(* Logix 5000 Rung export; software revision 16.03 *)

MODULES
   MNETC : vendor None type None code None
   Local : vendor None type None code None
END_MODULES

TYPE MNetCConnectionInput :
STRUCT
   Data : INT[62];   // Block Transfer Array Size [62] or [122] or [242]
END_STRUCT
END_TYPE

TYPE MNetCInitOutData :   // Used to bring the Module into a known state after a restart operation.
STRUCT
   InitOutBlkIDLim : INT;   // Block Index Limit for ReadData size of the array
END_STRUCT
END_TYPE

TYPE MnetCCmdControl :
STRUCT
   CmdCntReqClientID : INT;   // Block5000 Client IDentification by Index number 0 to 29
   CmdCntReqCMDqty : INT;   // Block5000 command quantity
   CmdCntReqCMDindex : INT[16];   // Contains index in the command list for the 1st command to be entered into Command queue
   WriteCmdBits : INT[30];   // This is for 30 Clients with 16 commands each.
   CmdBitsTrigger : BOOL;   // Activates the Selected Write Command Bits
END_STRUCT
END_TYPE

TYPE MNetCDATA :
STRUCT
   ReadData : INT[480];
   WriteData : INT[480];
END_STRUCT
END_TYPE

TYPE MNetCCONTROL :
STRUCT
   BootTimer : TIMER;
   ColdBoot : BOOL;   // Hardware reset of the Module
   WarmBoot : BOOL;   // Configuration data reset in the Module.
   EventCmd : MNetCEventCmd[1];
   EventCmdTrigger : BOOL;
   EventCmdPending : BOOL;   // Halts rung until Module is ready.
   CmdControl : MnetCCmdControl;
   CmdControlPending : BOOL;   // Halts rung until Module is ready.
   CmdControlTrigger : BOOL;
   IPAdressControl : MNetCIPAddress;
   CmdBitPending : BOOL;   // Halts rung until Module is ready.
   CmdBitTrigger : BOOL;
END_STRUCT
END_TYPE

TYPE MNetCCONFIG :
STRUCT
   BlockTransferSize : INT;   // Determines Register quantity to move across the Backplane
END_STRUCT
END_TYPE

TYPE MNetCIPAddress :   // Dynamicaly Alterable TCP/IP address for MNETC module. Block 9990 and 9991
STRUCT
   GetIPAddress : BOOL;   // Gets IP address
   GetIP : INT[4];   // Get IP
   GetIPAddressPending : BOOL;   // Halts rung until Module is ready.
   SetIPAddress : BOOL;   // Sets IP address
   SetIP : INT[4];   // Set IP
   SetIPAddrPending : BOOL;   // Halts rung until Module is ready.
   WriteIPAddressAck : INT[4];   // Module's response to Setting IP Address
END_STRUCT
END_TYPE

TYPE MNetCConnectionOutput :
STRUCT
   Data : INT[61];   // Block Transfer Array Size [61] or [121] or [241]
END_STRUCT
END_TYPE

TYPE MNetCSTATUS :   // This status data is returned on each read block and can be used to detect proper module operation.
STRUCT
   PassCnt : INT;   // Program cycle counter
   Block : MNetCBlockStats;   // Block transfer statistics
   MnetServer : MNetCPortStats;   // MNet server status data
   MBAPServer : MNetCPortStats;   // MBAP server status data
   StatReqClientID : INT;   // Block3000 Client IDentification by Index number 0 to 29
   CmdBits : INT[30];
   ClientStats : MNetCPortStats[30];   // Client status data
   ClientStatsPending : BOOL;   // Halts rung until Module is ready.
   ClientStatsTrigger : BOOL;   // Get Client Status
   CmdErrorList : INT[16];   // Cmd Error List
END_STRUCT
END_TYPE

TYPE MNetCModuleDef :
STRUCT
   CONFIG : MNetCCONFIG;
   DATA : MNetCDATA;
   CONTROL : MNetCCONTROL;
   STATUS : MNetCSTATUS;
   UTIL : MNetCUTIL;
END_STRUCT
END_TYPE

TYPE MNetCUTIL :
STRUCT
   ReadDataSizeGet : INT;   // Gets ReadData Array Length.
   WriteDataSizeGet : INT;   // Gets WriteData Array Length.
   ReadDataBlkCount : INT;   // holds the value of the Block Counts of the Read Data Array.
   WriteDataBlkCount : INT;   // holds the value of the Block Counts of the Write Data Array.
   RBTSremainder : INT;   // The remainder of the 60, 120 or 240 block to transfer.
   WBTSremainder : INT;   // The remainder of the 60, 120 or 240 block to transfer.
   LastRead : INT;   // Index of last read block
   LastWrite : INT;   // Index of last write block
   BlockIndex : INT;   // Computed block offset for data table
   StatusIndex : INT;   // Computed block offset for status data
   InitOutputData : MNetCInitOutData;
END_STRUCT
END_TYPE

TYPE MNetCPortStats :   // This object is used to store the port statistics for an MVI69-MNet port.
STRUCT
   CmdReq : INT;   // Total number of command list requests sent
   CmdResp : INT;   // Total number of command list responses received
   CmdErr : INT;   // Total number of command list errors
   Requests : INT;   // Total number of requests for port
   Responses : INT;   // Total number of responses for port
   ErrSent : INT;   // Total number of errors sent
   ErrRec : INT;   // Total number of errors received
   CfgErrWord : INT;   // Configuration Error Word
   CurErr : INT;   // Current Error code
   LastErr : INT;   // Last recorded error code
END_STRUCT
END_TYPE

TYPE MNetCBlockStats :   // This object is used to store the block transfer statistics for the MVI69-MNet module.
STRUCT
   Read : INT;   // Total number of read block transfers
   Write : INT;   // Total number of write block transfers
   Parse : INT;   // Total number of blocks parsed
   Event : INT;   // Total number of event blocks received
   Cmd : INT;   // Total number of command blocks received
   Err : INT;   // Total number of block transfer errors
END_STRUCT
END_TYPE

TYPE MNetCEventCmd :   // Data structure to use for Event message generation.
STRUCT
   IP0 : INT;   // TCP/IP-0 address for MNETC module
   IP1 : INT;   // TCP/IP-1 address for MNETC module
   IP2 : INT;   // TCP/IP-2 address for MNETC module
   IP3 : INT;   // TCP/IP-3 address for MNETC module
   ServPort : INT;   // TCP Service Port number (0-65535), 502 for MBAP, 2000 for MNET
   Node : INT;   // Modbus slave node address (0 to 247)
   DBAddress : INT;   // Module internal database to use with message
   Count : INT;   // Register or data point count
   Swap : INT;   // Swap code to use with functions 3 and 4
   Function : INT;   // Modbus function code for message
   Address : INT;   // Address to interface with in device
   EvntCmdClientID : INT;   // Block2000 Client IDentification by Index number 0 to 29
END_STRUCT
END_TYPE

ADD_ON_INSTRUCTION AOI69MNETC   (* revision 1.3, vendor ProSoft Technology Inc. *)
// Add On instruction interface between the CompactLogix backplane and the MVI69-MNETC module.
// Revision note:
// v1.3 - Initialize output data block now supports flexible read and write data array sizing.
VAR_IN_OUT
   Connection_Input : MNetCConnectionInput; {required}
   Connection_Output : MNetCConnectionOutput; {required}
   MNETC : MNetCModuleDef; {required}
END_VAR

ROUTINE Logic   (* ladder *)
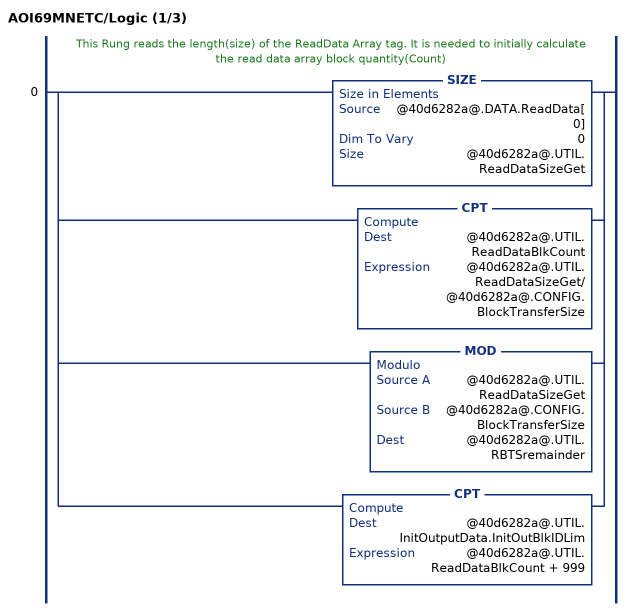
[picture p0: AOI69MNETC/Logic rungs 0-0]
   // This Rung reads the length(size) of the ReadData Array tag. It is needed to initially calculate the read data array block quantity(Count)
   0: [SIZE(@40d6282a@.DATA.ReadData[0],0,@40d6282a@.UTIL.ReadDataSizeGet) ,CPT(@40d6282a@.UTIL.ReadDataBlkCount,@40d6282a@.UTIL.ReadDataSizeGet/@40d6282a@.CONFIG.BlockTransferSize) ,MOD(@40d6282a@.UTIL.ReadDataSizeGet,@40d6282a@.CONFIG.BlockTransferSize,@40d6282a@.UTIL.RBTSremainder) ,CPT(@40d6282a@.UTIL.InitOutputData.InitOutBlkIDLim,@40d6282a@.UTIL.ReadDataBlkCount + 999) ];
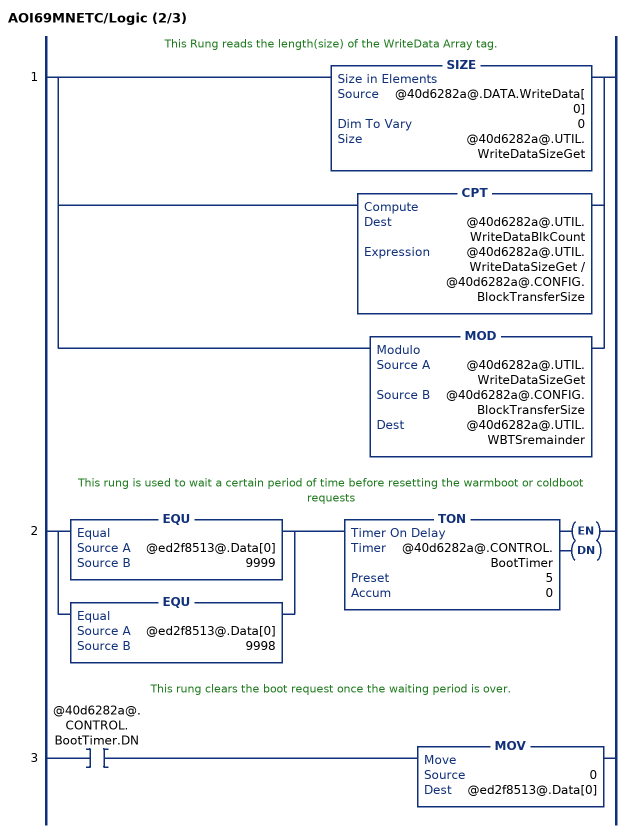
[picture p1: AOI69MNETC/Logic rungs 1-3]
   // This Rung reads the length(size) of the WriteData Array tag.
   1: [SIZE(@40d6282a@.DATA.WriteData[0],0,@40d6282a@.UTIL.WriteDataSizeGet) ,CPT(@40d6282a@.UTIL.WriteDataBlkCount,@40d6282a@.UTIL.WriteDataSizeGet / @40d6282a@.CONFIG.BlockTransferSize) ,MOD(@40d6282a@.UTIL.WriteDataSizeGet,@40d6282a@.CONFIG.BlockTransferSize,@40d6282a@.UTIL.WBTSremainder) ];
   // This rung is used to wait a certain period of time before resetting the warmboot or coldboot requests
   2: [EQU(@ed2f8513@.Data[0],9999) ,EQU(@ed2f8513@.Data[0],9998) ]TON(@40d6282a@.CONTROL.BootTimer,5,0);
   // This rung clears the boot request once the waiting period is over.
   3: XIC(@40d6282a@.CONTROL.BootTimer.DN)MOV(0,@ed2f8513@.Data[0]);
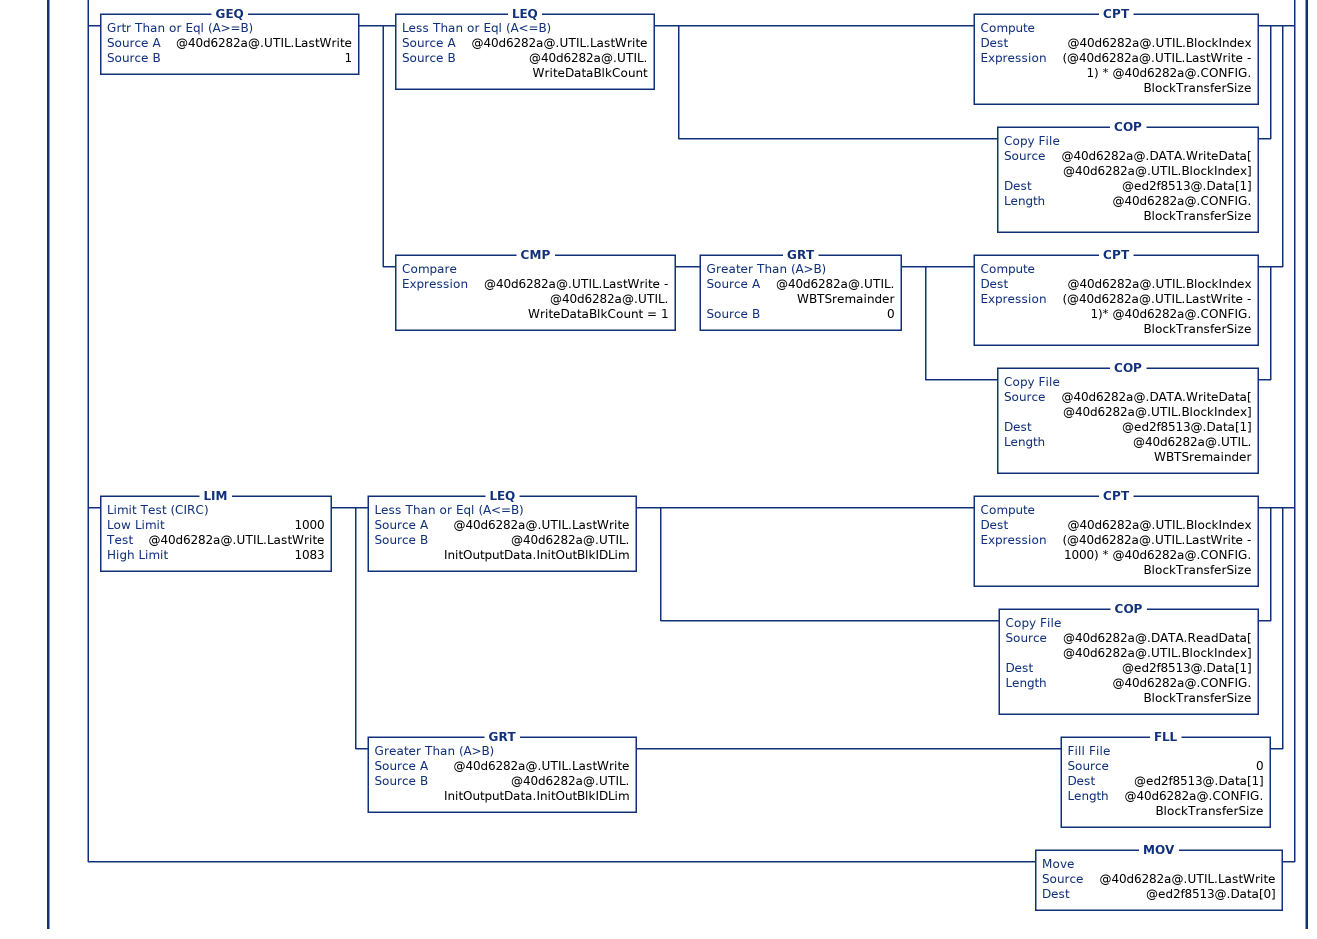
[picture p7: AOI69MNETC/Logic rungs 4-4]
   // This rung is used to check for a new read block from the MVI56-MNETC module in slot 1.  If new data is available, the LastRead and word[0] will not be equal.  This will force the program to call the ReadData subroutine to process the new data received.  After the new data is placed in the Modbus Data Table, the program will send new data to the module using the WriteData subroutine.
   4: NEQ(@f68caed0@.Data[0],@40d6282a@.UTIL.LastRead)[MOV(@f68caed0@.Data[0],@40d6282a@.UTIL.LastRead) ,GEQ(@40d6282a@.UTIL.LastRead,1) [LEQ(@40d6282a@.UTIL.LastRead,@40d6282a@.UTIL.ReadDataBlkCount) [CPT(@40d6282a@.UTIL.BlockIndex,(@40d6282a@.UTIL.LastRead-1)*@40d6282a@.CONFIG.BlockTransferSize) ,COP(@f68caed0@.Data[2],@40d6282a@.DATA.ReadData[@40d6282a@.UTIL.BlockIndex],@40d6282a@.CONFIG.BlockTransferSize) ] ,CMP(@40d6282a@.UTIL.LastRead - @40d6282a@.UTIL.ReadDataBlkCount = 1) GRT(@40d6282a@.UTIL.RBTSremainder,0) [CPT(@40d6282a@.UTIL.BlockIndex,(@40d6282a@.UTIL.LastRead - 1) * @40d6282a@.CONFIG.BlockTransferSize) ,COP(@f68caed0@.Data[2],@40d6282a@.DATA.ReadData[@40d6282a@.UTIL.BlockIndex],@40d6282a@.UTIL.RBTSremainder) ] ] ,[EQU(-1,@40d6282a@.UTIL.LastRead) ,EQU(0,@40d6282a@.UTIL.LastRead) ] [COP(@f68caed0@.Data[2],@40d6282a@.STATUS.PassCnt,1) ,COP(@f68caed0@.Data[3],@40d6282a@.STATUS.Block.Read,6) ,COP(@f68caed0@.Data[9],@40d6282a@.STATUS.CmdBits[0],30) ] ,LIM(2000,@40d6282a@.UTIL.LastRead,2029) EQU(@f68caed0@.Data[2],1) OTU(@40d6282a@.CONTROL.EventCmdPending) ,LIM(3000,@40d6282a@.UTIL.LastRead,3029) [COP(@f68caed0@.Data[2],@40d6282a@.STATUS.ClientStats[@40d6282a@.STATUS.StatReqClientID].CmdReq,10) ,COP(@f68caed0@.Data[12],@40d6282a@.STATUS.CmdErrorList[0],16) ,OTU(@40d6282a@.STATUS.ClientStatsPending) ] ,LIM(5000,@40d6282a@.UTIL.LastRead,5016) LIM(1,@f68caed0@.Data[2],16) OTU(@40d6282a@.CONTROL.CmdControlPending) ,EQU(@40d6282a@.UTIL.LastRead,9990) [COP(@f68caed0@.Data[2],@40d6282a@.CONTROL.IPAdressControl.WriteIPAddressAck[0],4) ,OTU(@40d6282a@.CONTROL.IPAdressControl.SetIPAddrPending) ] ,EQU(@40d6282a@.UTIL.LastRead,9991) [COP(@f68caed0@.Data[2],@40d6282a@.CONTROL.IPAdressControl.GetIP[0],4) ,OTU(@40d6282a@.CONTROL.IPAdressControl.GetIPAddressPending) ] ,MOV(@f68caed0@.Data[1],@40d6282a@.UTIL.LastWrite) ,LIM(1000,@40d6282a@.UTIL.LastWrite,1008) [CPT(@40d6282a@.UTIL.BlockIndex,(@40d6282a@.UTIL.LastWrite - 1000) * @40d6282a@.CONFIG.BlockTransferSize) ,COP(@40d6282a@.DATA.ReadData[@40d6282a@.UTIL.BlockIndex],@ed2f8513@.Data[1],@40d6282a@.CONFIG.BlockTransferSize) ] ,XIC(@40d6282a@.CONTROL.WarmBoot) [MOV(9998,@40d6282a@.UTIL.LastWrite) ,OTU(@40d6282a@.CONTROL.WarmBoot) ] ,XIC(@40d6282a@.CONTROL.ColdBoot) [MOV(9999,@40d6282a@.UTIL.LastWrite) ,OTU(@40d6282a@.CONTROL.ColdBoot) ] ,XIC(@40d6282a@.CONTROL.EventCmdTrigger) XIO(@40d6282a@.CONTROL.EventCmdPending) [COP(@40d6282a@.CONTROL.EventCmd[0].IP0,@ed2f8513@.Data[1],11) ,LIM(0,@40d6282a@.CONTROL.EventCmd[0].EvntCmdClientID,29) ADD(2000,@40d6282a@.CONTROL.EventCmd[0].EvntCmdClientID,@40d6282a@.UTIL.LastWrite) ,OTU(@40d6282a@.CONTROL.EventCmdTrigger) ,OTL(@40d6282a@.CONTROL.EventCmdPending) ] ,XIC(@40d6282a@.STATUS.ClientStatsTrigger) XIO(@40d6282a@.STATUS.ClientStatsPending) [LIM(0,@40d6282a@.STATUS.StatReqClientID,29) ADD(3000,@40d6282a@.STATUS.StatReqClientID,@40d6282a@.UTIL.LastWrite) ,OTL(@40d6282a@.STATUS.ClientStatsPending) ,OTU(@40d6282a@.STATUS.ClientStatsTrigger) ] ,XIC(@40d6282a@.CONTROL.CmdControlTrigger) XIO(@40d6282a@.CONTROL.CmdControlPending) [LIM(0,@40d6282a@.CONTROL.CmdControl.CmdCntReqClientID,29) MOV(@40d6282a@.CONTROL.CmdControl.CmdCntReqClientID,@ed2f8513@.Data[1]) ,COP(@40d6282a@.CONTROL.CmdControl.CmdCntReqCMDindex[0],@ed2f8513@.Data[2],16) ,LIM(1,@40d6282a@.CONTROL.CmdControl.CmdCntReqCMDqty,16) ADD(5000,@40d6282a@.CONTROL.CmdControl.CmdCntReqCMDqty,@40d6282a@.UTIL.LastWrite) ,OTL(@40d6282a@.CONTROL.CmdControlPending) ,OTU(@40d6282a@.CONTROL.CmdControlTrigger) ] ,[EQU(@40d6282a@.UTIL.LastWrite,0) ,EQU(@40d6282a@.UTIL.LastWrite,-1) ,XIC(@40d6282a@.CONTROL.CmdControl.CmdBitsTrigger) MOV(0,@40d6282a@.UTIL.LastWrite) ] [COP(@40d6282a@.CONTROL.CmdControl.WriteCmdBits[0],@ed2f8513@.Data[1],30) ,OTU(@40d6282a@.CONTROL.CmdControl.CmdBitsTrigger) ] ,XIC(@40d6282a@.CONTROL.IPAdressControl.SetIPAddress) XIO(@40d6282a@.CONTROL.IPAdressControl.SetIPAddrPending) [MOV(9990,@40d6282a@.UTIL.LastWrite) ,COP(@40d6282a@.CONTROL.IPAdressControl.SetIP[0],@ed2f8513@.Data[1],4) ,OTL(@40d6282a@.CONTROL.IPAdressControl.SetIPAddrPending) ,OTU(@40d6282a@.CONTROL.IPAdressControl.SetIPAddress) ] ,XIC(@40d6282a@.CONTROL.IPAdressControl.GetIPAddress) XIO(@40d6282a@.CONTROL.IPAdressControl.GetIPAddressPending) [MOV(9991,@40d6282a@.UTIL.LastWrite) ,OTL(@40d6282a@.CONTROL.IPAdressControl.GetIPAddressPending) ,OTU(@40d6282a@.CONTROL.IPAdressControl.GetIPAddress) ] ,GEQ(@40d6282a@.UTIL.LastWrite,1) [LEQ(@40d6282a@.UTIL.LastWrite,@40d6282a@.UTIL.WriteDataBlkCount) [CPT(@40d6282a@.UTIL.BlockIndex,(@40d6282a@.UTIL.LastWrite - 1) * @40d6282a@.CONFIG.BlockTransferSize) ,COP(@40d6282a@.DATA.WriteData[@40d6282a@.UTIL.BlockIndex],@ed2f8513@.Data[1],@40d6282a@.CONFIG.BlockTransferSize) ] ,CMP(@40d6282a@.UTIL.LastWrite - @40d6282a@.UTIL.WriteDataBlkCount = 1) GRT(@40d6282a@.UTIL.WBTSremainder,0) [CPT(@40d6282a@.UTIL.BlockIndex,(@40d6282a@.UTIL.LastWrite - 1)* @40d6282a@.CONFIG.BlockTransferSize) ,COP(@40d6282a@.DATA.WriteData[@40d6282a@.UTIL.BlockIndex],@ed2f8513@.Data[1],@40d6282a@.UTIL.WBTSremainder) ] ] ,LIM(1000,@40d6282a@.UTIL.LastWrite,1083) [LEQ(@40d6282a@.UTIL.LastWrite,@40d6282a@.UTIL.InitOutputData.InitOutBlkIDLim) [CPT(@40d6282a@.UTIL.BlockIndex,(@40d6282a@.UTIL.LastWrite - 1000) * @40d6282a@.CONFIG.BlockTransferSize) ,COP(@40d6282a@.DATA.ReadData[@40d6282a@.UTIL.BlockIndex],@ed2f8513@.Data[1],@40d6282a@.CONFIG.BlockTransferSize) ] ,GRT(@40d6282a@.UTIL.LastWrite,@40d6282a@.UTIL.InitOutputData.InitOutBlkIDLim) FLL(0,@ed2f8513@.Data[1],@40d6282a@.CONFIG.BlockTransferSize) ] ,MOV(@40d6282a@.UTIL.LastWrite,@ed2f8513@.Data[0]) ];
END_ROUTINE
END_ADD_ON_INSTRUCTION

VAR_GLOBAL   (* controller tags *)
   MNetC : MNetCModuleDef;
        .BP.LASTREAD   // this tag receives Block ID data from the last scan.
        .GETIPADDRESS   // Gets the IP address from the Module.
        .SETIPADDRESS   // Sets the IP address for the Module
   AOI69MNETC : AOI69MNETC;
   Local:1:I : AB:1769_MODULE_INT_128Bytes:I:0;
   Local:1:O : AB:1769_MODULE_INT_122Bytes:O:0;
   Connection_Output : MNetCConnectionOutput;
   Connection_Input : MNetCConnectionInput;
END_VAR

PROGRAM MainProgram

ROUTINE MainRoutine   (* ladder *)
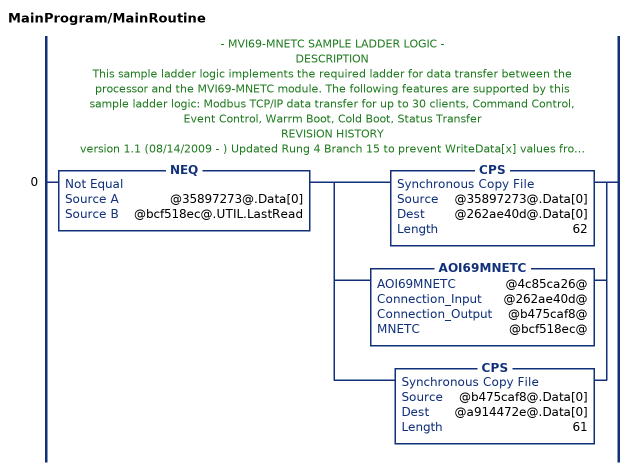
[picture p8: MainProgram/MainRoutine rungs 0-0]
   // - MVI69-MNETC SAMPLE LADDER LOGIC -
   // DESCRIPTION
   // This sample ladder logic implements the required ladder for data transfer between the processor and the MVI69-MNETC module. The following features are supported by this sample ladder logic: Modbus TCP/IP data transfer for up to 30 clients, Command Control, Event Control, Warrm Boot, Cold Boot, Status Transfer
   // REVISION HISTORY
   // version 1.1 (08/14/2009 - ) Updated Rung 4 Branch 15 to prevent WriteData[x] values from being applied as WriteCmdBits data when Block ID=0.
   // version 1.0. (08/29/2008) - Release
   0: NEQ(@35897273@.Data[0],@bcf518ec@.UTIL.LastRead)[CPS(@35897273@.Data[0],@262ae40d@.Data[0],62) ,AOI69MNETC(@4c85ca26@,@262ae40d@,@b475caf8@,@bcf518ec@) ,CPS(@b475caf8@.Data[0],@a914472e@.Data[0],61) ];
END_ROUTINE
END_PROGRAM
